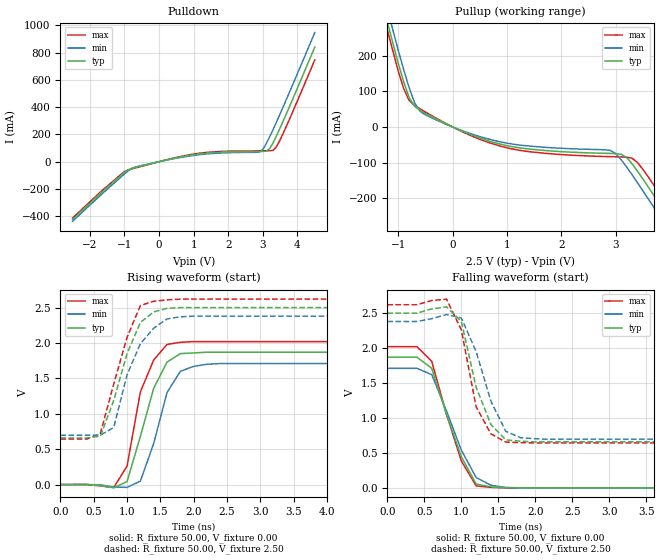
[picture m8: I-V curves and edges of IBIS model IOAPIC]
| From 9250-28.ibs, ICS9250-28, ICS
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|   Model IOAPIC
[Model]   IOAPIC
Model_type   Output
Polarity   Non-Inverting
Vmeas = 1.25V
Cref = 20pF
Rref = 0
Vref = 1.25V
C_comp   5.50pF   5.00pF   6.00pF
[Temperature Range]   27.00   70.00   0.00
[Voltage Range]   2.50V   2.38V   2.62V
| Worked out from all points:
|   slope of the pulldown table from 0 to 0.375 V, typ, clamps not added: 17 ohm
|   slope of the pullup table from 0 to 0.375 V, typ, clamps not added: 15.6 ohm
|   rising waveform, R_fixture 50.00, V_fixture 0.00: 20-80 % time 370ps typ, 335ps min, 309ps max; typ from 0 V to 1.87 V
|   rising waveform, R_fixture 50.00, V_fixture 2.50: 20-80 % time 392ps typ, 387ps min, 374ps max; typ from 0.659 V to 2.5 V
|   falling waveform, R_fixture 50.00, V_fixture 0.00: 20-80 % time 372ps typ, 404ps min, 343ps max; typ from 1.87 V to 0 V
|   falling waveform, R_fixture 50.00, V_fixture 2.50: 20-80 % time 302ps typ, 335ps min, 256ps max; typ from 2.5 V to 0.659 V
[Pulldown]
| voltage   I(typ)   I(min)   I(max)
-2.5V     -422mA     -436.9mA   -412.8mA
-1V       -77.23mA   -89.74mA   -71.79mA
-700mV    -43.7mA    -40.19mA   -47.17mA
1.1V      55.3mA     49.02mA    59.76mA
2.9V      75.02mA    70.77mA    79.41mA
3V        75.21mA    90.56mA    79.57mA
3.1V      76.93mA    132.5mA    79.73mA
3.2V      96.86mA    183.4mA    79.96mA
3.3V      140.6mA    237.8mA    83.53mA
3.4V      192.8mA    294.2mA    112.5mA
3.7V      363.1mA    468.3mA    271.4mA
4.5V      839.9mA    946.2mA    745.7mA
[Pullup]
| voltage   I(typ)   I(min)   I(max)
-2.5V     1.06A      1.1A       1.04A
-1.6V     525mA      563mA      501.4mA
-1V       178.9mA    215.4mA    157mA
-800mV    82.92mA    110.6mA    74.57mA
-600mV    46.69mA    44.18mA    50.74mA
400mV     -25.58mA   -22.22mA   -28.47mA
1.3V      -60.1mA    -51.95mA   -67.19mA
2.9V      -74.41mA   -65.84mA   -83.39mA
3.3V      -103.2mA   -133.9mA   -87.74mA
3.9V      -238.5mA   -272.6mA   -209.2mA
4.2V      -309.6mA   -343.7mA   -280mA
4.5V      -381.3mA   -415.4mA   -351.7mA
[Ramp]
| variable   typ   min   max
dV/dt_r   1.12/255.91p   1.02/287.43p   1.21/235.57p
dV/dt_f   1.10/200.00p   1.01/300.00p   1.18/200.00p
[Rising Waveform]
R_fixture = 50.00
V_fixture = 0.00
V_fixture_min = 0.00
V_fixture_max = 0.00
| time   V(typ)   V(min)   V(max)
0s        0V         0V         0V
800ps     -46.73mV   -35.18mV   -42.06mV
1ns       42.27mV    -40.23mV   261.1mV
1.2ns     680.7mV    48.69mV    1.31V
1.4ns     1.36V      581mV      1.76V
1.6ns     1.73V      1.3V       1.98V
1.8ns     1.85V      1.6V       2.01V
2ns       1.86V      1.67V      2.02V
2.4ns     1.87V      1.71V      2.02V
10ns      1.87V      1.71V      2.02V
[Rising Waveform]
R_fixture = 50.00
V_fixture = 2.50
V_fixture_min = 2.38
V_fixture_max = 2.62
| time   V(typ)   V(min)   V(max)
0s        659mV      696.6mV    643.4mV
400ps     658.9mV    696.5mV    643.1mV
600ps     683.7mV    697.8mV    724.4mV
800ps     1.19V      806.1mV    1.42V
1ns       1.85V      1.55V      2.08V
1.2ns     2.29V      1.99V      2.53V
1.4ns     2.44V      2.21V      2.59V
1.6ns     2.49V      2.34V      2.61V
2ns       2.5V       2.38V      2.62V
10ns      2.5V       2.38V      2.62V
[Falling Waveform]
R_fixture = 50.00
V_fixture = 0.00
V_fixture_min = 0.00
V_fixture_max = 0.00
| time   V(typ)   V(min)   V(max)
0s        1.87V      1.71V      2.02V
400ps     1.87V      1.71V      2.02V
600ps     1.71V      1.62V      1.81V
800ps     1.05V      1.1V       1.05V
1ns       445.7mV    539.2mV    384.7mV
1.2ns     54.46mV    148.1mV    28.42mV
1.4ns     13.33mV    37.09mV    6.94mV
1.6ns     1.4mV      5.89mV     781.1uV
1.8ns     511.8uV    1.12mV     249.3uV
10ns      1.54uV     1.66uV     0V
[Falling Waveform]
R_fixture = 50.00
V_fixture = 2.50
V_fixture_min = 2.38
V_fixture_max = 2.62
| time   V(typ)   V(min)   V(max)
0s        2.5V       2.38V      2.62V
400ps     2.5V       2.38V      2.62V
800ps     2.59V      2.48V      2.7V
1ns       2.38V      2.43V      2.26V
1.2ns     1.44V      1.95V      1.16V
1.4ns     906.3mV    1.24V      772.2mV
1.6ns     686mV      809.6mV    654.9mV
1.8ns     666.8mV    717.6mV    646.6mV
2.2ns     658.7mV    695.3mV    643.1mV
10ns      659mV      696.6mV    643.4mV
